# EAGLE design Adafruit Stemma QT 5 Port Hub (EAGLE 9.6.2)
COMPANY: ADAFRUIT INDUSTRIES; DRAWN: KTOWN; REV: A
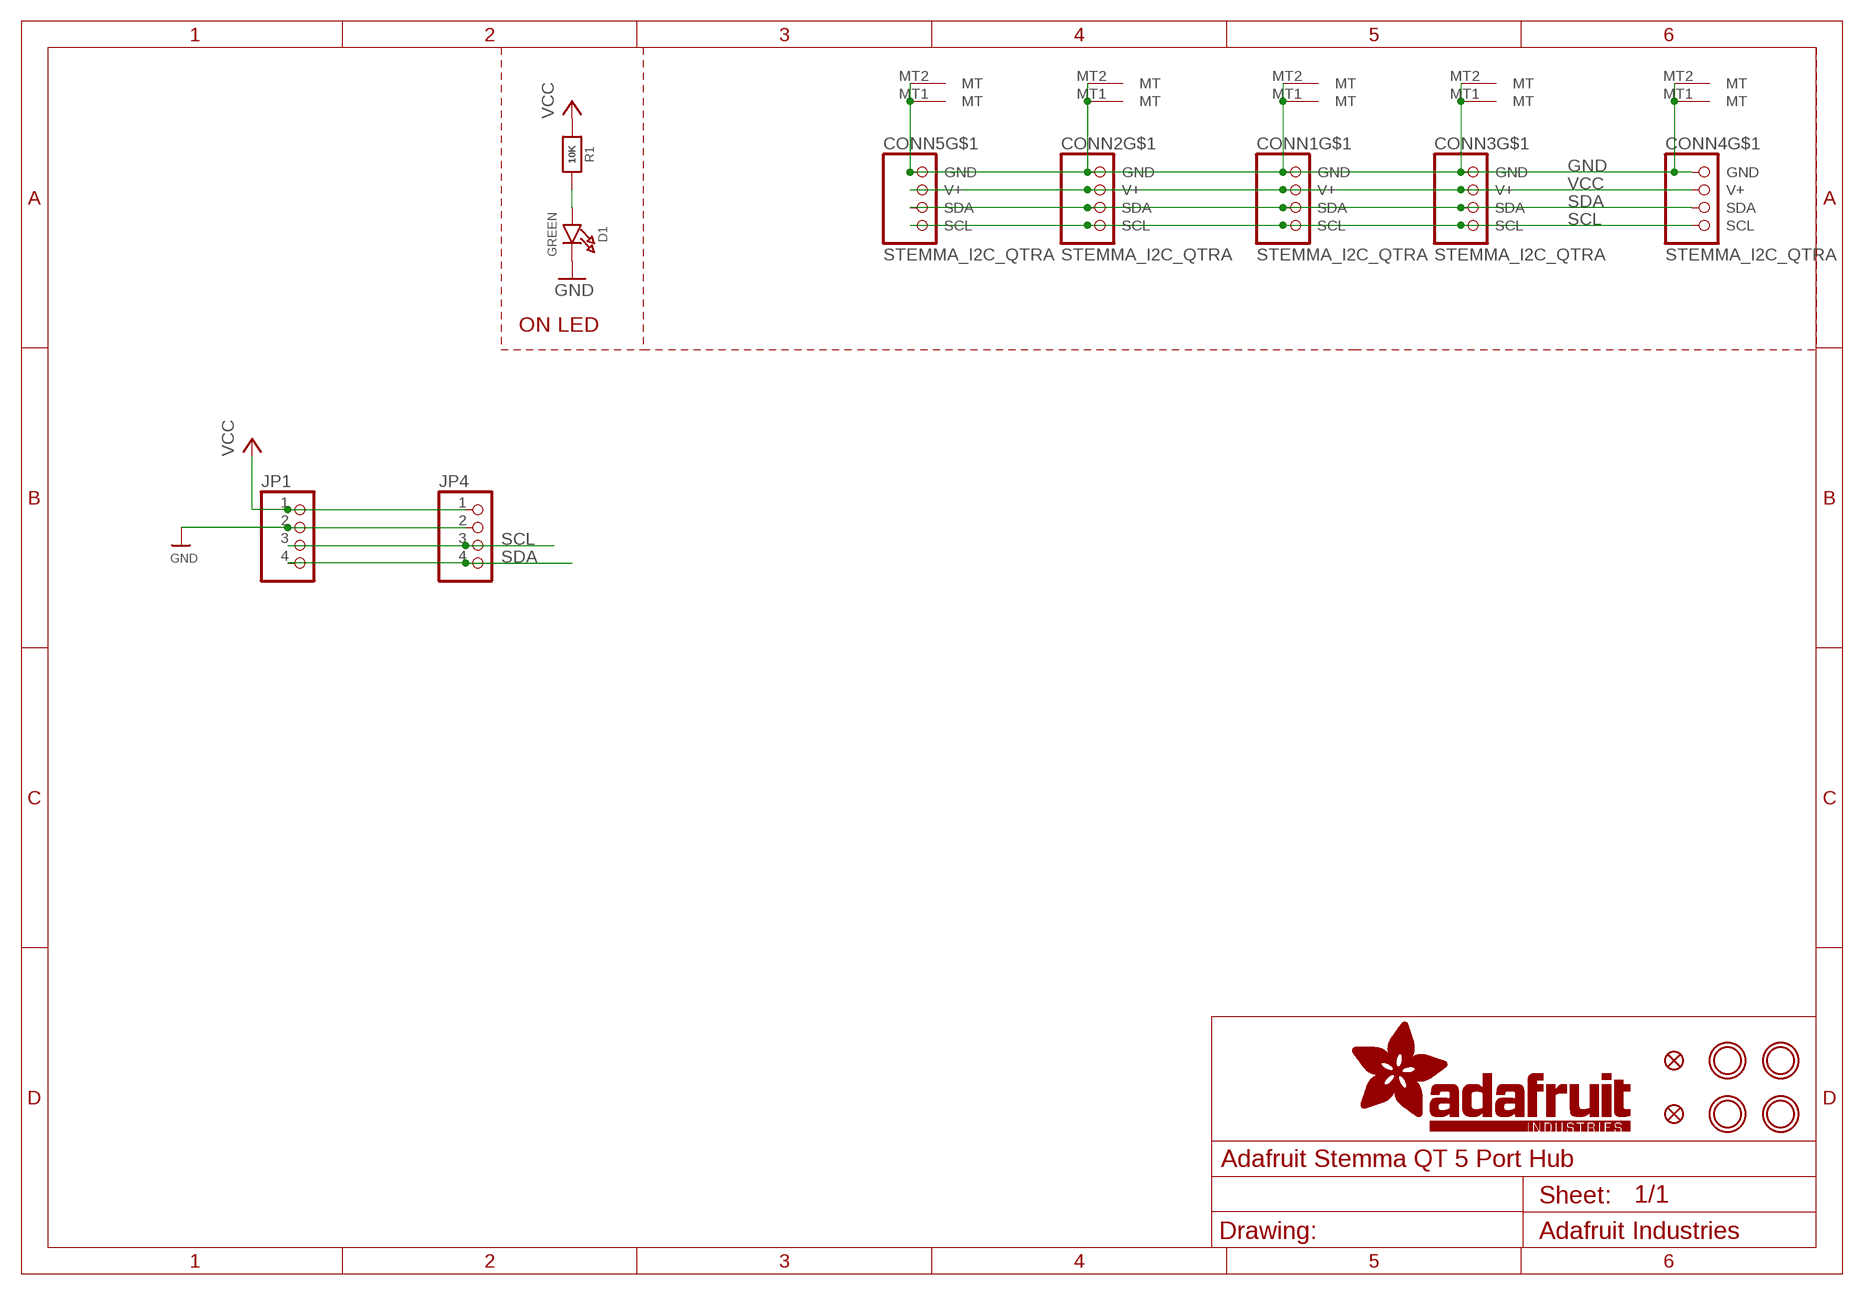
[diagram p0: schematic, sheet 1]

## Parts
CONN1  STEMMA_I2C_QTRA  [JST_SH4_RA]
CONN2  STEMMA_I2C_QTRA  [JST_SH4_RA]
CONN3  STEMMA_I2C_QTRA  [JST_SH4_RA]
CONN4  STEMMA_I2C_QTRA  [JST_SH4_RA]
CONN5  STEMMA_I2C_QTRA  [JST_SH4_RA]
D1  GREEN  LED0603_NOOUTLINE  [CHIPLED_0603_NOOUTLINE]
FID3  FIDUCIAL_1MM  [FIDUCIAL_1MM]
FID4  FIDUCIAL_1MM  [FIDUCIAL_1MM]
JP1  HEADER-1X476MIL  [1X04_ROUND_76]
JP4  HEADER-1X476MIL  [1X04_ROUND_76]
R1  10K  RESISTOR_0603_NOOUT  [0603-NO]
U$1  MOUNTINGHOLE2.5  [MOUNTINGHOLE_2.5_PLATED]
U$17  MOUNTINGHOLE2.5  [MOUNTINGHOLE_2.5_PLATED]
U$19  MOUNTINGHOLE2.5  [MOUNTINGHOLE_2.5_PLATED]
U$21  MOUNTINGHOLE2.5  [MOUNTINGHOLE_2.5_PLATED]

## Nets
GND [highpower]: CONN1.1(GND) CONN1.MT1(MT) CONN1.MT2(MT) CONN2.1(GND) CONN2.MT1(MT) CONN2.MT2(MT) CONN3.1(GND) CONN3.MT1(MT) CONN3.MT2(MT) CONN4.1(GND) CONN4.MT1(MT) CONN4.MT2(MT) CONN5.1(GND) CONN5.MT1(MT) CONN5.MT2(MT) D1.C JP1.2 JP4.2
N$1: D1.A R1.2
SCL: CONN1.4(SCL) CONN2.4(SCL) CONN3.4(SCL) CONN4.4(SCL) CONN5.4(SCL) JP1.3 JP4.3
SDA: CONN1.3(SDA) CONN2.3(SDA) CONN3.3(SDA) CONN4.3(SDA) CONN5.3(SDA) JP1.4 JP4.4
VCC [highpower]: CONN1.2(V+) CONN2.2(V+) CONN3.2(V+) CONN4.2(V+) CONN5.2(V+) JP1.1 JP4.1 R1.1

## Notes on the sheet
- ON LED

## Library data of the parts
CONN1-CONN5 = adafruit_electromech:STEMMA_I2C; LCSC: C145961
D1 = microbuilder:LED: LED; JLC_ROTATION: 270
FID3 FID4 = microbuilder:FIDUCIAL: Fiducial Alignment Points; BOM: EXCLUDE
JP1 JP4 = microbuilder:HEADER-1X4: PIN HEADER
R1 = microbuilder:RESISTOR: Resistors
U$1 U$17 U$19 U$21 = microbuilder:MOUNTINGHOLE: Mounting Hole; BOM: EXCLUDE

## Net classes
1 highpower: width 0.305 mm, drill 0.483 mm
2 lowpower: width 0.254 mm, drill 0.483 mm

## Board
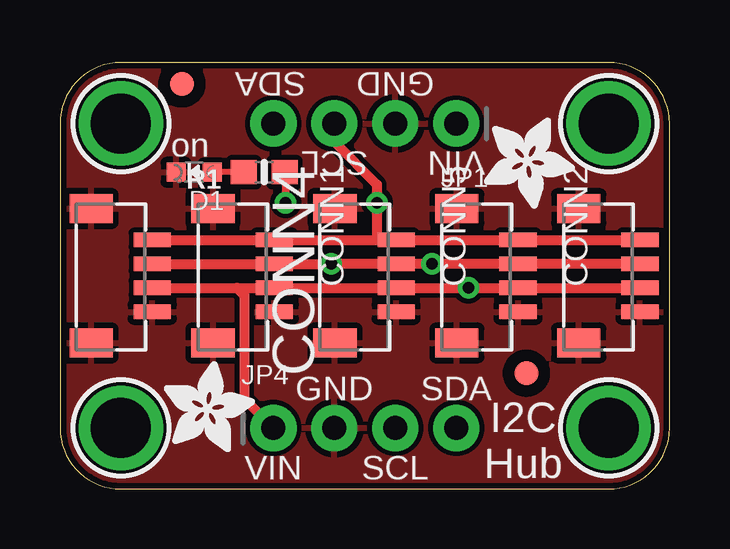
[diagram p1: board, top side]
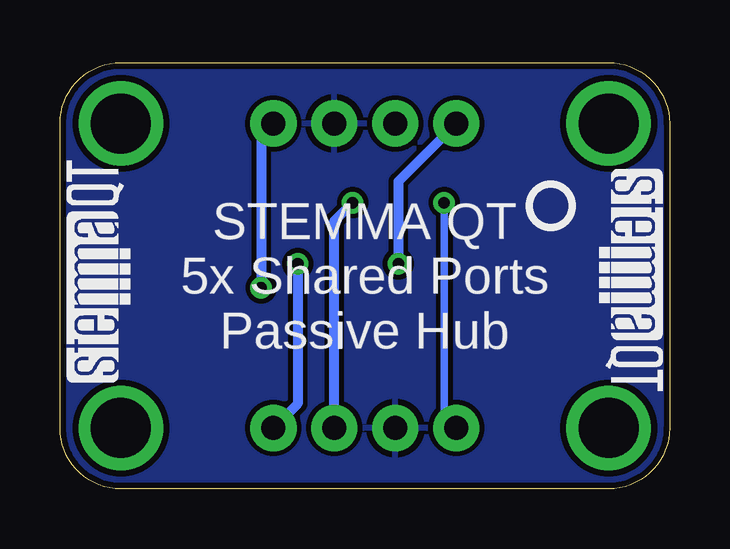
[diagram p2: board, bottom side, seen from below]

Size 25.4 x 17.78 mm. Coordinates in mm from the lower left corner, seen from the top.
Outline: 0,15.24 0,2.54 arc90 2.54,0 22.86,0 arc90 25.4,2.54 25.4,15.24 arc90 22.86,17.78 2.54,17.78 arc90 0,15.24
Copper layers (1*16): Top 0.035mm / dielectric 1.5mm / Bottom 0.035mm
Design rules "adafruit *": minimum track width 8mil, minimum drill 15.5mil, track to track 8mil, track to pad 8mil, pad to pad 8mil, via to via 8mil, smd to smd 8mil, copper to edge 10mil, drill to drill 8mil, minimum pad ring 10mil, minimum via ring 8mil, stop-mask expansion 2mil, vias tented up to drill 20mil, thermal gap 10mil

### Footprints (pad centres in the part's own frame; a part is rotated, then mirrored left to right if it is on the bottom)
JST_SH4_RA = smd 0.6 x 1.55: 1 1.5,0.924; 2 0.5,0.924; 3 -0.5,0.924; 4 -1.5,0.924 | smd 1.2 x 1.8: MT1 -2.8,-1.624; MT2 2.8,-1.624
CHIPLED_0603_NOOUTLINE = smd 0.8 x 0.8: A 0,-0.75; C 0,0.75
FIDUCIAL_1MM = smd 1 x 1: 1 0,0
1X04_ROUND_76 = drill 1 pad 1.93: 1 -3.81,0; 2 -1.27,0; 3 1.27,0; 4 3.81,0
0603-NO = smd 1.075 x 1: 1 -0.85,0; 2 0.85,0
MOUNTINGHOLE_2.5_PLATED = drill 2.5 pad 3.2: P$1 0,0

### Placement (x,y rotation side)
CONN1  8,8.89 270 top
CONN2  18.16,8.89 270 top
CONN3  23.24,8.89 270 top
CONN4  2.92,8.89 270 top
CONN5  13.08,8.89 270 top
D1  5.59,13.21 90 top
FID3  19.43,4.83 0 top
FID4  5.08,16.89 0 top
JP1  12.7,15.24 180 top
JP4  12.7,2.54 0 top
R1  8.51,13.21 180 top
U$1  2.54,15.24 0 top
U$2  [ADAFRUIT_3.5MM]  4.32,1.52 0 top
U$3  [ADAFRUIT_3.5MM]  17.65,15.49 270 top
U$17  22.86,15.24 0 top
U$19  2.54,2.54 0 top
U$21  22.86,2.54 0 top
U$25  [PCBFEAT-REV-040]  4.95,11.81 0 bottom
U$30  [STEMMAQT]  22.48,4.45 90 bottom
U$31  [STEMMAQT]  2.92,13.34 270 bottom

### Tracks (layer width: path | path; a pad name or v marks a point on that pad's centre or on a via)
GND
  pour Top: 0,17.78 25.4,17.78 25.4,0 0,0
  pour Bottom: 0,17.78 25.4,17.78 25.4,0 0,0
N$1
  Top 0.254: R1.2 D1.A
SCL  (via drill 0.48)
  Top 0.406: CONN4.4 CONN1.4 13.21,10.39 | 13.21,10.39 CONN5.4 CONN2.4 CONN3.4 | JP1.3 11.43,14.48 13.21,12.7 v13.21,11.94 13.21,10.39
  Bottom 0.406: JP4.3 13.97,11.18 v13.21,11.94
SDA  (via drill 0.48)
  Top 0.406: CONN3.3 CONN2.3 v15.49,9.39 CONN5.3 v11.3,9.39 CONN1.3 CONN4.3
  Bottom 0.406: JP1.4 11.3,12.83 v11.3,9.39 | v15.49,9.39 15.49,3.56 JP4.4
VCC  (via drill 0.48)
  Top 0.305: v9.4,11.94 9.4,13.17 R1.1
  Top 0.406: CONN4.2 7.37,8.39 | 7.37,8.39 CONN1.2 CONN5.2 | CONN5.2 14.47,8.39 14.48,8.38 | CONN5.2 v17.02,8.39 CONN2.2 CONN3.2 | 7.37,8.39 7.68,8.07 7.68,3.75 JP4.1
  Bottom 0.305: v9.4,11.94 9.4,3.05 JP4.1
  Bottom 0.406: JP1.1 17.02,14.73 v17.02,8.39

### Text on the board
tPlace: SDA | GND | on | SCL | VIN | GND | SDA | I2C / Hub | VIN | SCL
bPlace: STEMMA QT / 5x Shared Ports / Passive Hub

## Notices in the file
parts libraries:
microbuilder: This work is placed in the public domain, and may be freely used for commercial and non-commercial work with the following conditions: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
